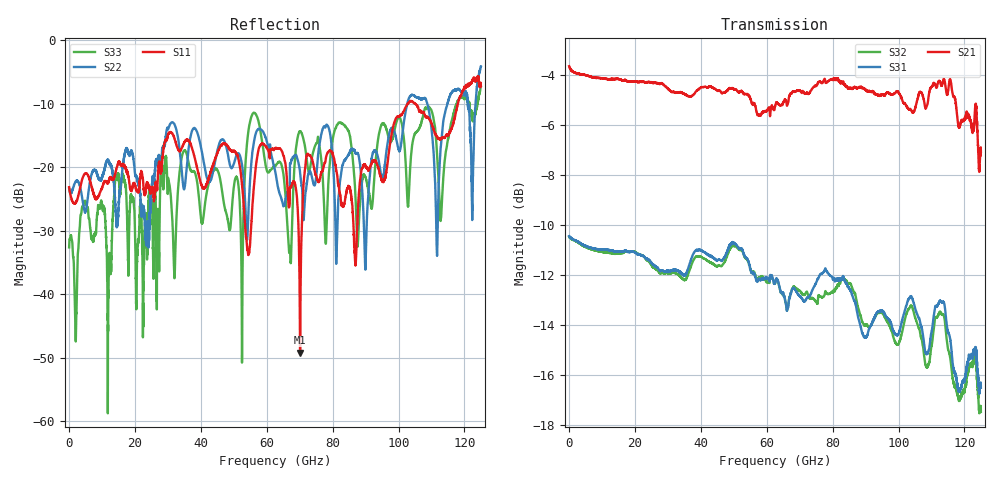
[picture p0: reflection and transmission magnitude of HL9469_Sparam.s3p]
! 5/10/2023 4:11:25 PM
! H:\PROTOTYPE_DATA\110GHZ-POT\A-3PORT\S21.S3P
! CHANNEL.1
! TR.MEASUREMENT
! CORRECTED.DATA
! RF.CORRECTION: FULL.TWO.PORT.CAL.PORT.1.2
! AVERAGING: 1 PointByPoint
! IF.BANDWIDTH: 1KHZ
! SWEEPTYPE:  FREQ.SWEEP(Linear)
! Reference Plane Port Info
! PORT:  PORT1  PORT2
! DISTANCE:  0  m  0  m
! TIME:  0  s  0  s
! PHASE.OFFSET:  0 °  0 °
! LOSS:  0  dB  0  dB
! REF.LOSS:  0  dB  0  dB
! REF.FREQ:  0  Hz  0  Hz
! Power Info
! POWER:  -10  dBm  -10  dBm
! EFF.POWER:  -10  dBm  -10  dBm
! POWER(>54G):  -10  dBm  -10  dBm
! EFF.POWER(>54G):  -10  dBm  -10  dBm
! SOURCE.ATTEN:  0  dB  0  dB
! TEST.ATTEN:  0  dB  0  dB
# GHZ S RI R 50.0
! FREQ.GHZ S11RE S11IM S12RE S12IM S13RE S13IM
! S21RE S21IM S22RE S22IM S23RE S23IM
! S31RE S31IM S32RE S32IM S33RE S33IM
!; PortSelection: Port_123
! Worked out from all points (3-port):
!   5000 points, 25 MHz to 125 GHz, reference 50 ohm
!   strongest paths, dB at 25 MHz, 31.27 GHz, 62.52 GHz, 93.78 GHz, 125 GHz:
!     S21: -3.6, -4.7, -5.2, -4.8, -7.1
!     S31: -10.4, -11.8, -12.3, -13.5, -16.5
!     S32: -10.5, -11.9, -12.3, -13.5, -17.5
!   lowest |S11| = -49.2 dB at 70.12 GHz (marker M1), VSWR 1.01, Z = 50.3 - j0.0457 ohm
!   |S11| at or under -10 dB: start of sweep to 102.8 GHz; 105.1 GHz to 118 GHz (12.91 GHz wide, 11.6 % of centre)
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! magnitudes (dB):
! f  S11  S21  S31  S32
! 25 MHz  -23.1  -3.6  -10.4  -10.5
! 54.42 GHz  -33.7  -4.8  -11.4  -11.5
! 62.52 GHz  -17.0  -5.2  -12.3  -12.3
! 67.03 GHz  -23.2  -4.8  -12.9  -12.9
! 70.12 GHz  -49.2  -4.6  -12.8  -12.6
! 72.5 GHz  -17.9  -4.7  -12.9  -12.8
! 89.95 GHz  -19.9  -4.6  -14.5  -14.0
! 107.8 GHz  -11.5  -5.1  -14.8  -15.2
! 111.7 GHz  -15.2  -4.5  -13.3  -13.7
! 125 GHz  -7.2  -7.1  -16.5  -17.5
